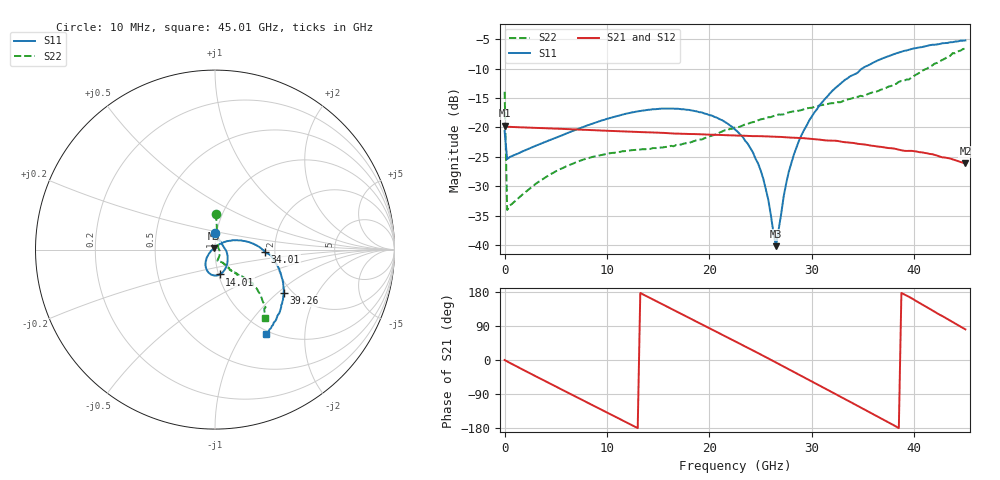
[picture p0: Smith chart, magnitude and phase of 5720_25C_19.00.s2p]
! Device:  ADRF5720
! Description: 0.5dB LSB GaAs MMIC 6-bit Digital Attenuator
! Frequency:  0.000009 -  40 GHz
! Ports:
!	RF1	= Port 1
!	RF2	= Port 2
! Vdd:  3.3 Volt
! Vss:  -3.3 Volt
! Control:  0/3.3 Volt
! State:  19.00 dB attenuation
! Data:  The device was measured using G-S-G Probes on a matrix board.
!  Data was collected using an calibrated 4 port network analyzer.
!  The reference plane for this measurement is at the launchers.
! Note:  Analog Devices supplies this data as a sample of measured data
!  for this product.  Your particular data for this product may vary.
!  Data was taken at 25 degrees C.
!  Analog Devices reserves the right to change this data at anytime.
# GHZ S DB R 45.0
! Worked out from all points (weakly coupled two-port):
!   181 points, 10 MHz to 45.01 GHz, reference 45 ohm
!   highest |S21| = -19.70 dB at 10 MHz (marker M1); lowest = -26.1 dB at 45.01 GHz (marker M2)
!   lowest |S11| = -40.2 dB at 26.51 GHz (marker M3), VSWR 1.02, Z = 44.4 + j0.622 ohm
!   |S11| at or under -10 dB: start of sweep to 34.92 GHz
!   |S22| runs from -34.0 to -6.5 dB; largest |S21 - S12| = 0.00014
!   S11 on the Smith chart (normalised r, x): 10 MHz: 0.98, +0.18; 14.01 GHz: 1.01, -0.29; 34.01 GHz: 1.77, -0.05; 39.26 GHz: 1.81, -1.09; 45.01 GHz: 0.95, -1.28
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0.01  -20.61 90.6  -19.70 -0.1  -19.70 -0.2  -13.94 88.6
0.26  -25.38 8.9  -19.89 -3.9  -19.90 -3.9  -34.05 24.3
3.26  -22.97 -18.0  -20.09 -45.9  -20.09 -45.8  -29.33 -37.8
7.76  -19.87 -47.5  -20.40 -107.8  -20.40 -107.8  -25.44 -69.6
14.01  -17.01 -79.4  -20.84 166.5  -20.84 166.5  -23.65 -75.9
15.26  -16.81 -85.3  -20.92 149.2  -20.91 149.2  -23.43 -73.7
19.26  -17.45 -105.1  -21.18 94.2  -21.18 94.2  -22.07 -62.3
22.76  -20.72 -125.3  -21.39 45.9  -21.39 46.0  -19.98 -55.6
24.01  -23.51 -134.7  -21.47 28.7  -21.47 28.7  -19.21 -54.7
25.01  -27.27 -144.2  -21.49 14.7  -21.49 14.7  -18.63 -54.3
25.76  -32.29 -160.7  -21.54 4.1  -21.54 4.1  -18.28 -54.0
26.51  -40.20 134.2  -21.60 -6.5  -21.60 -6.4  -17.97 -54.2
27.26  -31.78 64.6  -21.65 -17.3  -21.65 -17.2  -17.78 -53.1
27.76  -27.56 49.9  -21.71 -24.2  -21.72 -24.1  -17.45 -53.1
28.76  -22.24 36.2  -21.80 -38.4  -21.80 -38.4  -17.16 -53.4
30.26  -17.46 23.2  -22.00 -60.0  -22.00 -60.0  -16.52 -52.5
32.01  -13.79 10.7  -22.26 -84.8  -22.26 -84.8  -15.88 -51.5
34.01  -11.11 -2.8  -22.63 -114.2  -22.63 -114.2  -15.02 -47.7
37.76  -7.70 -24.1  -23.54 -168.3  -23.55 -168.2  -12.96 -43.9
39.26  -6.91 -32.2  -24.00 170.3  -24.00 170.2  -11.86 -44.0
42.26  -5.88 -46.9  -24.80 123.2  -24.79 123.1  -9.01 -44.7
45.01  -5.21 -59.0  -26.11 80.8  -26.11 80.9  -6.54 -53.5
